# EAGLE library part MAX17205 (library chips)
Stand-Alone ModelGauge m5 Fuel Gauge with SHA-256 Authentication
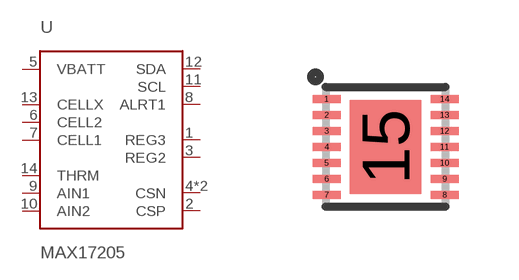
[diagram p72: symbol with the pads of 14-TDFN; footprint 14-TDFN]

Designator prefix U

## MAX17205 (MOUSER: 700-MAX17205G+00E)  [14-TDFN]
1  REG3
2  CSP
3  REG2
4  CSN
5  VBATT
6  CELL2
7  CELL1
8  ALRT1
9  AIN1
10  AIN2
11  SCL
12  SDA
13  CELLX
14  THRM
15  CSN

## Footprint 14-TDFN (pad centres in mm)
smd 0.7 x 0.2: 1 -1.475,1.2; 2 -1.475,0.8; 3 -1.475,0.4; 4 -1.475,0; 5 -1.475,-0.4; 6 -1.475,-0.8; 7 -1.475,-1.2; 8 1.475,-1.2; 9 1.475,-0.8; 10 1.475,-0.4; 11 1.475,0; 12 1.475,0.4; 13 1.475,0.8; 14 1.475,1.2
smd 1.78 x 2.35: 15 0,0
